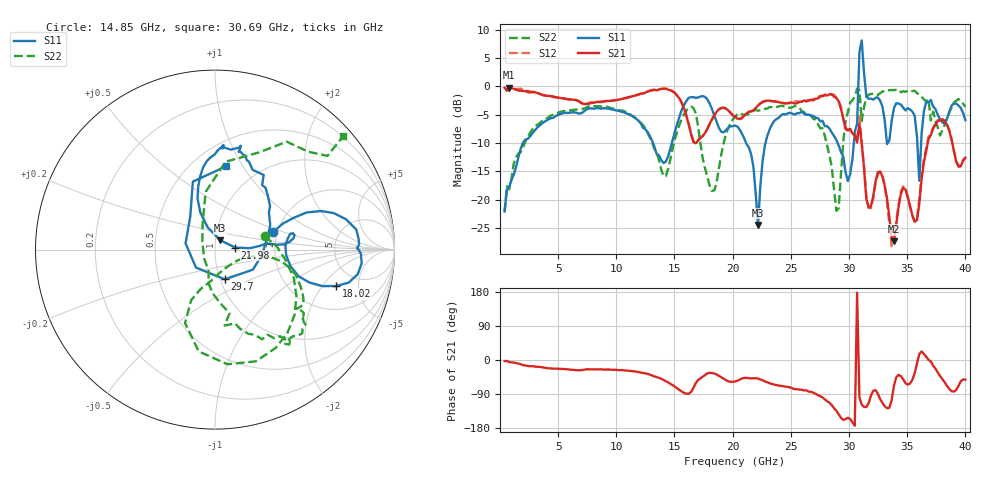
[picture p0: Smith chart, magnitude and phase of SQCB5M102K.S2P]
! Network Analyzer HP8722ES.07.66: Jul 25, 2000 Serial No. US39175408
! 27 Oct 2004  15:13:28
! Frequency  S11  S21  S12  S22
# HZ  S  DB R  50
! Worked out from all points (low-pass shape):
!   201 points, 400 MHz to 40 GHz, reference 50 ohm
!   highest |S21| = -0.22 dB at 796 MHz (marker M1); lowest = -27.4 dB at 33.86 GHz (marker M2)
!   |S21| within 3 dB of the highest: start of sweep to 15.69 GHz; 22.27 GHz to 29.19 GHz (6.925 GHz wide, 26.9 % of centre)
!   lowest |S11| = -24.5 dB at 22.18 GHz (marker M3), VSWR 1.13, Z = 52.6 + j5.58 ohm
!   |S11| at or under -10 dB: start of sweep to 1.969 GHz; 13.15 GHz to 14.78 GHz (1.624 GHz wide, 11.6 % of centre); 21.15 GHz to 22.82 GHz (1.669 GHz wide, 7.59 % of centre)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
!   |S22| runs from -22.1 to -0.4 dB; largest |S21 - S12| = 0.1
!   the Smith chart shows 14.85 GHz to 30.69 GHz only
!   S11 on the Smith chart (normalised r, x): 14.85 GHz: 1.90, +0.42; 18.02 GHz: 3.43, -2.76; 21.98 GHz: 1.25, +0.03; 29.7 GHz: 1.05, -0.36; 30.69 GHz: 0.71, +0.84
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4e8  -22.09 -103.5  -0.25 -2.7  -0.19 -2.3  -22.15 -105.4
7.96e8  -17.75 -79.7  -0.22 -5.4  -0.34 -4.8  -18.20 -99.3
7.132e9  -4.59 -88.3  -3.05 -26.3  -3.16 -26.9  -3.98 -133.1
1.3666e10  -12.19 -50.6  -0.57 -47.0  -0.51 -46.9  -12.99 142.9
1.4854e10  -9.40 17.0  -0.90 -66.7  -0.85 -67.0  -10.84 15.1
1.8022e10  -3.04 -16.7  -6.60 -33.7  -6.68 -34.1  -17.51 -79.2
2.02e10  -6.93 10.4  -5.37 -56.7  -5.36 -56.5  -5.40 -25.4
2.1982e10  -18.98 6.0  -3.85 -48.2  -3.83 -48.3  -4.18 -37.5
2.218e10  -24.46 62.0  -3.39 -49.0  -3.38 -48.9  -4.29 -37.5
2.3368e10  -6.75 98.4  -2.63 -63.2  -2.62 -63.2  -3.67 -40.6
2.6932e10  -5.22 71.9  -2.49 -86.2  -2.29 -88.1  -5.73 -66.1
2.8912e10  -9.46 23.9  -2.04 -133.9  -2.05 -134.9  -22.00 -138.8
2.9704e10  -15.18 -71.7  -7.55 -155.8  -7.35 -156.6  -6.15 83.2
3.0694e10  -6.61 82.6  -9.92 177.6  -9.73 177.5  -0.40 41.5
3.0892e10  6.06 39.5  -6.67 -98.5  -4.97 -99.1  -0.67 -110.1
3.109e10  8.11 -74.1  -10.04 -118.0  -10.01 -120.4  -6.11 -26.6
3.1486e10  -1.76 -61.8  -19.88 -124.3  -19.50 -129.2  -1.83 1.3
3.3466e10  -9.58 -84.7  -23.11 -126.0  -24.25 -124.4  -0.69 -6.6
3.3862e10  -3.84 -87.3  -27.36 -67.9  -27.57 -59.9  -0.67 -10.9
3.604e10  -16.69 -101.2  -20.71 15.8  -19.83 20.1  -1.47 -32.1
3.7624e10  -5.03 -104.4  -6.06 -32.9  -5.97 -33.0  -7.24 -44.7
4e10  -5.97 -97.0  -12.62 -52.0  -12.52 -50.6  -3.62 -43.7
